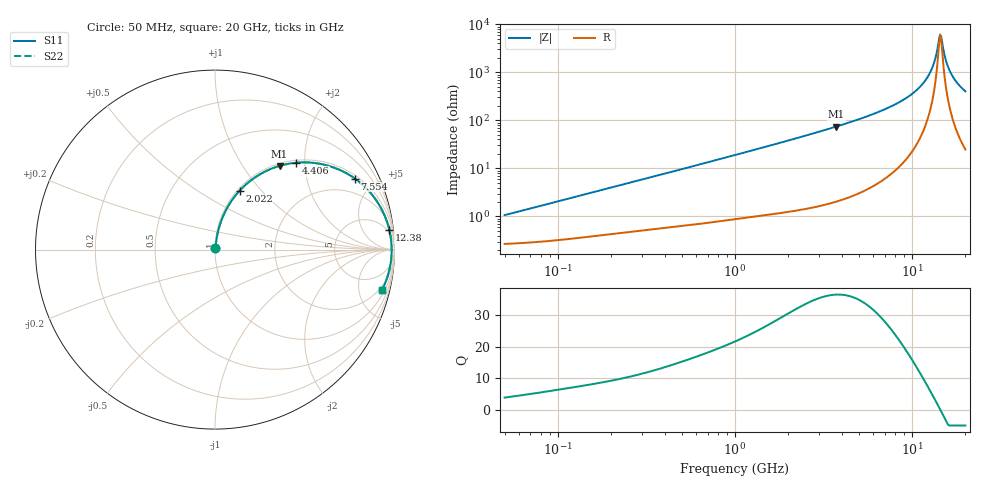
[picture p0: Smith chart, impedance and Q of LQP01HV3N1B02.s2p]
!Murata Part Number: LQP01HV3N1B02
!These Parameters are Measured in Series Mode Connection
!  o--[Z]--o
!Port1  Port2
!  o-------o
!Freq. Start=50[MHz] Stop=20[GHz], 401[Steps]
# Hz S RI R 50
!Freq.(Hz) S11(Real) S11(Imag) S21(Real) S21(Imag) S12(Real) S12(Imag) S22(Real) S22(Imag)
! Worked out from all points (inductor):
!   401 points, 50 MHz to 20 GHz, reference 50 ohm
!   read as one part in series: L = 3.27 nH near 51.52 MHz
!   highest Q = 36.6 at 3.736 GHz (marker M1), where L = 3.17 nH
!   self-resonance near 14.39 GHz
!   S11 on the Smith chart (normalised r, x): 50 MHz: 1.01, +0.02; 2.022 GHz: 1.03, +0.77; 4.406 GHz: 1.05, +1.80; 7.554 GHz: 1.15, +3.85; 12.38 GHz: 3, +17; 20 GHz: 1.50, -8.04
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5e7  0.00277 0.0102  0.9972 -0.0102  0.9972 -0.0102  0.00277 0.0102
1.364002e8  0.00436 0.0272  0.9956 -0.0272  0.9956 -0.0272  0.00436 0.0272
3.721004e8  0.0106 0.0709  0.9894 -0.0709  0.9894 -0.0709  0.0106 0.0709
1e9  0.0425 0.18  0.9575 -0.18  0.9575 -0.18  0.0425 0.18
2.021818e9  0.1369 0.3279  0.8631 -0.3279  0.8631 -0.3279  0.1369 0.3279
2.728004e9  0.2236 0.4024  0.7764 -0.4024  0.7764 -0.4024  0.2236 0.4024
3.736399e9  0.3598 0.4665  0.6402 -0.4665  0.6402 -0.4665  0.3598 0.4665
4.405649e9  0.4498 0.4838  0.5502 -0.4838  0.5502 -0.4838  0.4498 0.4838
5.769027e9  0.615 0.4715  0.385 -0.4715  0.385 -0.4715  0.615 0.4715
7.442007e9  0.7706 0.4018  0.2294 -0.4018  0.2294 -0.4018  0.7706 0.4018
7.554318e9  0.7791 0.3959  0.2209 -0.3959  0.2209 -0.3959  0.7791 0.3959
1.019291e10  0.9201 0.24  0.0799 -0.24  0.0799 -0.24  0.9201 0.24
1.131968e10  0.9523 0.1719  0.0477 -0.1719  0.0477 -0.1719  0.9523 0.1719
1.238412e10  0.9712 0.1099  0.0288 -0.1099  0.0288 -0.1099  0.9712 0.1099
1.314879e10  0.9793 0.0674  0.0207 -0.0674  0.0207 -0.0674  0.9793 0.0674
1.417136e10  0.984 0.0134  0.016 -0.0134  0.016 -0.0134  0.984 0.0134
1.438523e10  0.9842 0.0026  0.0158 -0.0026  0.0158 -0.0026  0.9842 0.0026
1.482269e10  0.9839 -0.0191  0.0161 0.0191  0.0161 0.0191  0.9839 -0.0191
1.550395e10  0.9817 -0.0515  0.0183 0.0515  0.0183 0.0515  0.9817 -0.0515
1.646126e10  0.9754 -0.0944  0.0246 0.0944  0.0246 0.0944  0.9754 -0.0944
1.800918e10  0.9589 -0.1573  0.0411 0.1573  0.0411 0.1573  0.9589 -0.1573
2e10  0.9295 -0.227  0.0705 0.227  0.0705 0.227  0.9295 -0.227
